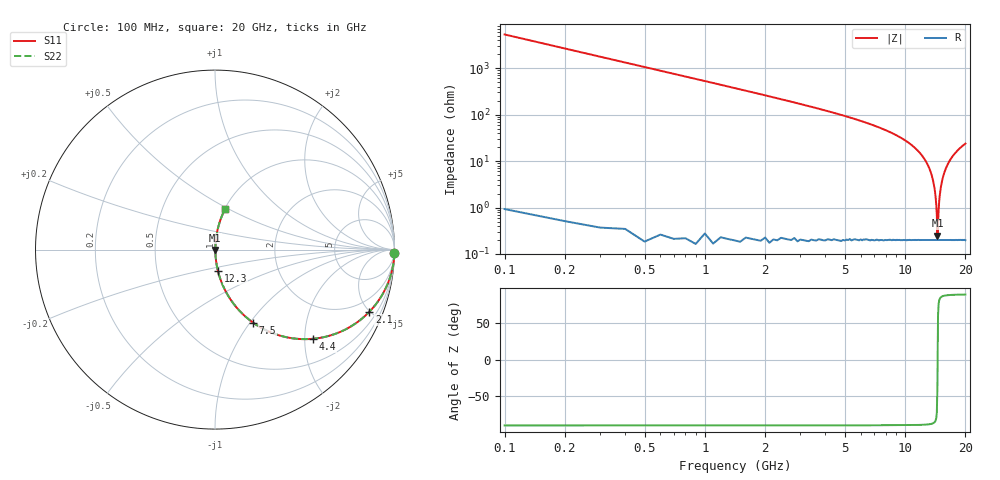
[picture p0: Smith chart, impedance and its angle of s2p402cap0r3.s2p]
! AVX Thin Film Operation		Date: April 2003
! Description: Accu-P® Series, Thin Film, SMD, RF Capacitor
! Part Number: 04023J0R3ABW
! 50 MHz  -  20 GHz
! Serial Measurements
# hz S db R 50
!	S11		S21		S12		S22
!	dB	Phase	dB	Phase	dB	Phase	dB	Phase
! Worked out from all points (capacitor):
!   200 points, 100 MHz to 20 GHz, reference 50 ohm
!   read as one part in series: C = 300 fF near 200 MHz
!   lowest |Z| = 247 mohm at 14.5 GHz (marker M1)
!   series resonance near 14.53 GHz, so ESL is about 400 pH
!   S11 on the Smith chart (normalised r, x): 100 MHz: open; 2.1 GHz: 1.00, -4.95; 4.4 GHz: 1.00, -2.19; 7.5 GHz: 1.00, -1.04; 12.3 GHz: 1.00, -0.24; 20 GHz: 1.00, +0.48
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1e8  -0.00 -1.1  -34.50 88.9  -34.50 88.9  -0.00 -1.1
2e8  -0.01 -2.2  -28.48 87.8  -28.48 87.8  -0.01 -2.2
3e8  -0.01 -3.2  -24.96 86.8  -24.96 86.8  -0.01 -3.2
7e8  -0.08 -7.5  -17.65 82.5  -17.65 82.5  -0.08 -7.5
1.3e9  -0.26 -13.9  -12.40 76.1  -12.40 76.1  -0.26 -13.9
2.1e9  -0.66 -22.0  -8.53 68.0  -8.53 68.0  -0.66 -22.0
3.5e9  -1.74 -35.0  -4.83 54.9  -4.83 54.9  -1.74 -35.0
4.4e9  -2.64 -42.4  -3.43 47.5  -3.43 47.5  -2.64 -42.4
6.8e9  -5.69 -58.5  -1.38 31.3  -1.38 31.3  -5.69 -58.5
7.5e9  -6.75 -62.4  -1.05 27.4  -1.05 27.4  -6.75 -62.4
1.01e10  -11.65 -74.4  -0.32 15.2  -0.32 15.2  -11.65 -74.4
1.23e10  -18.34 -82.1  -0.08 7.0  -0.08 7.0  -18.34 -82.1
1.34e10  -24.59 -84.7  -0.03 3.4  -0.03 3.4  -24.59 -84.7
1.39e10  -29.82 -84.6  -0.02 1.8  -0.02 1.8  -29.82 -84.6
1.42e10  -35.49 -82.2  -0.02 1.0  -0.02 1.0  -35.49 -82.2
1.44e10  -43.36 -72.5  -0.02 0.4  -0.02 0.4  -43.36 -72.5
1.45e10  -52.16 -35.8  -0.02 0.1  -0.02 0.1  -52.16 -35.8
1.48e10  -37.31 80.8  -0.02 -0.8  -0.02 -0.8  -37.31 80.8
1.51e10  -31.00 84.3  -0.02 -1.6  -0.02 -1.6  -31.00 84.3
1.57e10  -24.96 84.7  -0.03 -3.2  -0.03 -3.2  -24.96 84.7
1.67e10  -19.88 83.1  -0.06 -5.8  -0.06 -5.8  -19.88 83.1
2e10  -12.74 76.2  -0.25 -13.3  -0.25 -13.3  -12.74 76.2
